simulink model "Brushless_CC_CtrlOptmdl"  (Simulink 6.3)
settings: Solver=ode3  StartTime=0.0  StopTime=30.0  FixedStep=1e-3  MaxStep=1e-6  MinStep=1e-6  RelTol=1e-6  AbsTol=1e-6
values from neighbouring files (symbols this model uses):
  b = 0.8*Nm*s/rad    (= 0.8)    [Brushless_CC_CtrlOpt.m]
  Cr = 0*N*m    (= 0)    [Brushless_CC_CtrlOpt.m]
  Imax = 5.6*Amp    (= 5.6)    [Brushless_CC_CtrlOpt.m]
  J = 8*kg*m^2    (= 8)    [Brushless_CC_CtrlOpt.m]
  K = acker(A,B,lambda_alt)    [Brushless_CC_CtrlOpt.m]
  Ke = 10*N*m/Amp    (= 10)    [Brushless_CC_CtrlOpt.m]
  Kups = -inv(C(1:2)*inv(A(1:2,1:2)+B(1:2)*K(1:2))*B(1:2))    [Brushless_CC_CtrlOpt.m]
  La = 0.1*Henry    (= 0.1)    [Brushless_CC_CtrlOpt.m]
  Ra = 8*Ohm    (= 8)    [Brushless_CC_CtrlOpt.m]

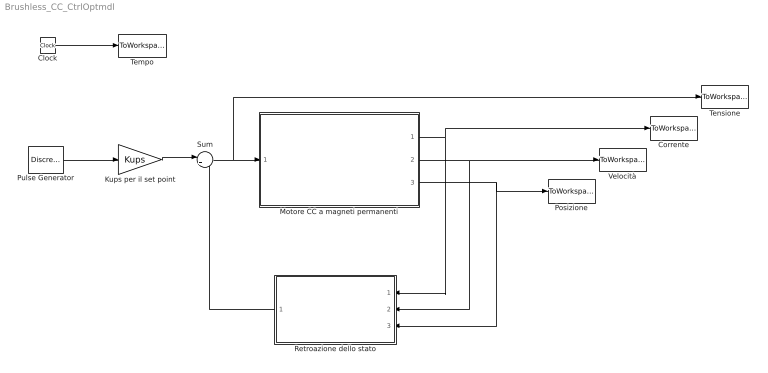
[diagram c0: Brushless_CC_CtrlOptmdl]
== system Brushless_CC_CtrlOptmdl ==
  Clock : Clock
  Corrente : ToWorkspace  VariableName=I  SampleTime=-1  SaveFormat=Array
  Kups per il set point : Gain  Gain=Kups  Multiplication=Matrix(K*u)
  Motore CC a magneti permanenti : Subsystem
  Posizione : ToWorkspace  VariableName=theta  SampleTime=-1  SaveFormat=Array
  Pulse Generator : DiscretePulseGenerator  PulseType=Time based  Amplitude=3  Period=6  PulseWidth=50
  Retroazione dello stato : Subsystem  Orientation=left
  Sum : Sum  Inputs=|++
  Tempo : ToWorkspace  VariableName=time  SampleTime=-1  SaveFormat=Array
  Tensione : ToWorkspace  VariableName=V  SampleTime=-1  SaveFormat=Array
  Velocità : ToWorkspace  VariableName=omega  SampleTime=-1  SaveFormat=Array
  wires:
  Motore CC a magneti permanenti/2(Velocità) -> Retroazione dello stato/2(Velocità), Velocità/1
  Motore CC a magneti permanenti/1(Corrente I) -> Retroazione dello stato/1(Corrente), Corrente/1
  Motore CC a magneti permanenti/3(Posizione  angolare) -> Posizione/1, Retroazione dello stato/3(Posizione  angolare)
  Clock/1 -> Tempo/1
  Retroazione dello stato/1(Retroazione) -> Sum/2
  Sum/1 -> Motore CC a magneti permanenti/1(Tensione V), Tensione/1
  Kups per il set point/1 -> Sum/1
  Pulse Generator/1 -> Kups per il set point/1

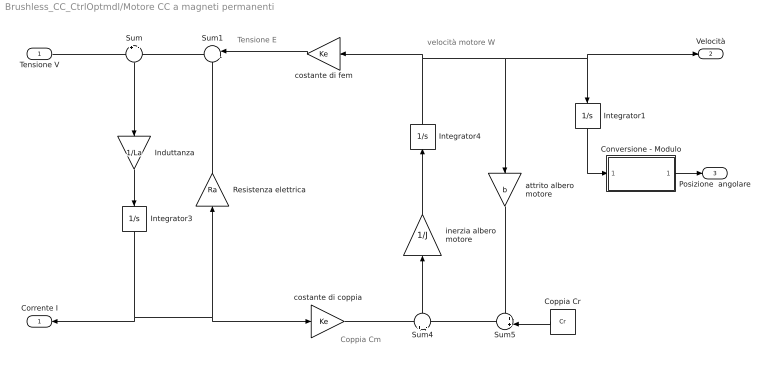
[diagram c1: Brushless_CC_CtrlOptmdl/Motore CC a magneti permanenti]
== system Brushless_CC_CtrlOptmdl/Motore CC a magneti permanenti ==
  note: Coppia Cm
  note: velocità motore W
  note: Tensione E
  Tensione V : Inport
  Conversione - Modulo : Subsystem
  Coppia Cr : Constant  Orientation=left  Value=Cr
  Induttanza : Gain  Orientation=down  Gain=1/La
  Integrator1 : Integrator  Orientation=down
  Integrator3 : Integrator  Orientation=down  LimitOutput=on  UpperSaturationLimit=Imax  LowerSaturationLimit=-Imax
  Integrator4 : Integrator  Orientation=up
  Resistenza elettrica : Gain  Orientation=up  Gain=Ra
  Sum : Sum  Orientation=down  Inputs=+|-
  Sum1 : Sum  Orientation=left  Inputs=|++
  Sum4 : Sum  Orientation=up  Inputs=+|-
  Sum5 : Sum  Orientation=left  Inputs=++|
  attrito albero motore : Gain  Orientation=down  Gain=b
  costante di coppia : Gain  Gain=Ke
  costante di fem : Gain  Orientation=left  Gain=Ke
  inerzia albero motore : Gain  Orientation=up  Gain=1/J
  Corrente I : Outport  Orientation=left
  Velocità : Outport  Port=2
  Posizione  angolare : Outport  Port=3
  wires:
  Integrator4/1 -> costante di fem/1, Integrator1/1, Velocità/1, attrito albero motore/1
  Integrator3/1 -> Resistenza elettrica/1, costante di coppia/1, Corrente I/1
  Tensione V/1 -> Sum/1
  Sum/1 -> Induttanza/1
  Induttanza/1 -> Integrator3/1
  Resistenza elettrica/1 -> Sum1/2
  Sum4/1 -> inerzia albero motore/1
  inerzia albero motore/1 -> Integrator4/1
  Sum5/1 -> Sum4/2
  attrito albero motore/1 -> Sum5/1
  costante di fem/1 -> Sum1/1
  Coppia Cr/1 -> Sum5/2
  Sum1/1 -> Sum/2
  costante di coppia/1 -> Sum4/1
  Conversione - Modulo/1(gradi) -> Posizione  angolare/1
  Integrator1/1 -> Conversione - Modulo/1(radianti)

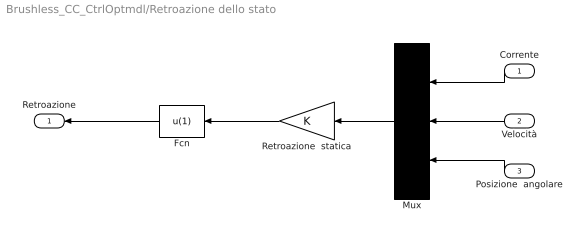
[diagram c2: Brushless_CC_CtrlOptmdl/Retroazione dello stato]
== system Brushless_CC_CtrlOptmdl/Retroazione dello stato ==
  Corrente : Inport  Orientation=left
  Velocità : Inport  Orientation=left  Port=2
  Posizione  angolare : Inport  Orientation=left  Port=3
  Fcn : Fcn  Orientation=left  Expr=u(1)
  Mux : Mux  Orientation=left  Inputs=3
  Retroazione  statica : Gain  Orientation=left  Gain=K  Multiplication=Matrix(K*u)
  Retroazione : Outport  Orientation=left
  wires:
  Mux/1 -> Retroazione  statica/1
  Retroazione  statica/1 -> Fcn/1
  Corrente/1 -> Mux/1
  Velocità/1 -> Mux/2
  Posizione  angolare/1 -> Mux/3
  Fcn/1 -> Retroazione/1

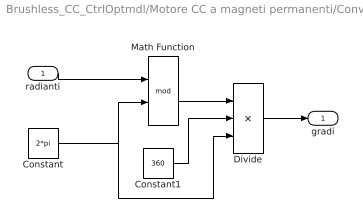
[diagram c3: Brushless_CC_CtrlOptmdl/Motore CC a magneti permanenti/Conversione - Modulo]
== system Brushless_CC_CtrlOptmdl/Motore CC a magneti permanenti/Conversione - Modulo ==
  radianti : Inport
  Constant : Constant  Value=2*pi
  Constant1 : Constant  Value=360
  Divide : Product  Inputs=**/  OutScaling=2^-10
  Math Function : Math  Operator=mod
  gradi : Outport
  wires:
  Math Function/1 -> Divide/1
  Constant1/1 -> Divide/2
  radianti/1 -> Math Function/1
  Constant/1 -> Divide/3, Math Function/2
  Divide/1 -> gradi/1
